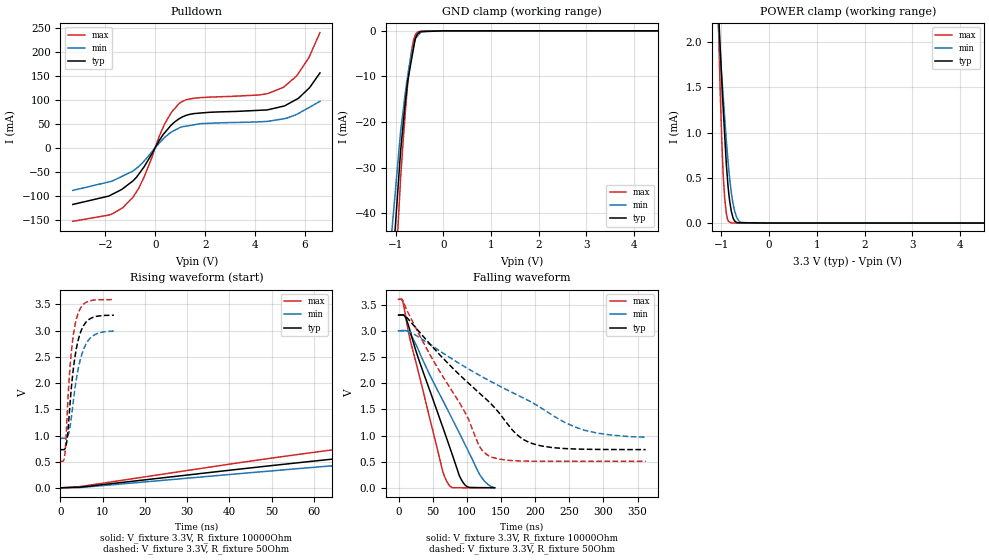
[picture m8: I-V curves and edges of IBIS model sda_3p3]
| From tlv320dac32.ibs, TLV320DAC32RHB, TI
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|   sda_3p3 Model
[Model]   sda_3p3
Model_type   I/O_open_drain
Polarity   Inverting
Vinl = 0.99
Vinh = 2.31
Vmeas = 1.65
Vref = 3.3
Cref = 10pF
Rref = 10000
|   typ   min   max
|   (nom PVT)   (fast PVT)   (slow PVT)
|C_comp from frequency sweep method (F=0.4MHz)
|C_comp   2.677e-10   2.502e-10   2.745e-10
|ON state : BUFFER OUTPUT TURNED LOW
|C_comp   5.318e-10   4.968e-10   5.453e-10
|OFF state: BUFFER IN HIGH IMPEDANCE
|C_comp   3.566e-12   3.518e-12   3.605e-12
|C_comp from LC tank measurement(L=1nH)
|Resonant Frequency(Hz)   4.560e+09   4.570e+09   4.560e+09
|C_comp   1.219e-12   1.214e-12   1.219e-12
|ON state : BUFFER OUTPUT TURNED LOW
|Resonant Frequency(Hz)   4.560e+09   4.570e+09   4.560e+09
|C_comp   1.219e-12   1.214e-12   1.219e-12
|OFF state: BUFFER IN HIGH IMPEDANCE
|Resonant Frequency(Hz)   4.780e+09   4.800e+09   4.770e+09
C_comp   1.110e-12   1.100e-12   1.114e-12
[model spec]
|subparameter   typ   min   max
Vinl   0.99   0.90   1.08
Vinh   2.31   2.10   2.52
| Where nom  PVT is Nominal Process, 3.3V, 45C
|   Fast PVT is Strong Process,  3.6V, -40C
|   Slow PVT is Weak Process,   3V, 105C
[Voltage Range]   3.3   3   3.6
|Ambient Temperature   25   85   -40
|Junction Temperature
[Temperature Range]   45   105   -40
[Pullup Reference]   3.3   3   3.6
[Pulldown Reference]   0   0   0
[Power Clamp Reference]   3.3   3   3.6
[GND Clamp Reference]   0   0   0
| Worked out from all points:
|   slope of the pulldown table from 0 to 0.495 V, typ, clamps not added: 13 ohm
|   GND clamp passes 1 mA (typ) near -0.56 V on its own axis
|   POWER clamp passes 1 mA (typ) near -0.93 V on its own axis
|   falling waveform, V_fixture 3.3V, R_fixture 10000Ohm: 20-80 % time 53.1ns typ, 68.9ns min, 41.1ns max; typ from 3.3 V to 0.004 V
|   rising waveform, V_fixture 3.3V, R_fixture 10000Ohm: 20-80 % time 454ns typ, 534ns min, 373ns max; typ from 0.003 V to 3.3 V
|   falling waveform, V_fixture 3.3V, R_fixture 50Ohm: 20-80 % time 115ns typ, 164ns min, 79.8ns max; typ from 3.3 V to 0.731 V
|   rising waveform, V_fixture 3.3V, R_fixture 50Ohm: 20-80 % time 2.17ns typ, 2.62ns min, 1.74ns max; typ from 0.731 V to 3.29 V
[Pulldown]
|   Voltage   I(typ)   I(min)   I(max)
-3.3V     -118.5mA   -89.27mA   -153.7mA
-1.696V   -96.69mA   -69.08mA   -137.7mA
-896.4mV  -69.64mA   -49.05mA   -103.7mA
-439.2mV  -39.66mA   -27.69mA   -60.66mA
381.6mV   31.19mA    21.56mA    49.68mA
1.001V    61.54mA    42.22mA    93.59mA
1.591V    71.25mA    47.97mA    103.4mA
4.162V    77.88mA    53.87mA    109.8mA
5.137V    86.55mA    60.08mA    125.8mA
5.674V    101.1mA    69.49mA    150.1mA
6.152V    123.6mA    83.47mA    187.5mA
6.6V      156mA      96.54mA    240.1mA
[GND Clamp]
|   Voltage   I(typ)   I(min)   I(max)
-3.3V     -1.343A    -1.199A    -1.533A
-1.487V   -114.4mA   -92.2mA    -146.8mA
-897.6mV  -26.39mA   -22.11mA   -32.41mA
-792mV    -15.05mA   -13.04mA   -16.99mA
-745.8mV  -10.84mA   -9.703mA   -11.43mA
-702mV    -8.268mA   -6.817mA   -7.045mA
-622.8mV  -3.616mA   -3.166mA   -1.957mA
-590.7mV  -1.731mA   -1.919mA   -1.015mA
-532.8mV  -615uA     -1.015mA   -208.3uA
-465mV    -195.4uA   -194.6uA   -64.22uA
-285mV    -119.2uA   -2.502uA   -4.665uA
6.6V      0A         0A         0A
[POWER Clamp]
|   Voltage   I(typ)   I(min)   I(max)
-3.3V     32.08mA    22.4mA     56.05mA
-1.089V   2.679mA    2.39mA     2.744mA
-1.03V    1.983mA    1.906mA    1.532mA
-993.6mV  1.586mA    1.634mA    934uA
-964.8mV  1.288mA    1.419mA    561.5uA
-932.4mV  983.8uA    1.176mA    280.4uA
-896.4mV  648.9uA    907.5uA    104uA
-864.6mV  429.3uA    705.3uA    36.05uA
-792mV    130.4uA    335uA      1.308uA
-681mV    8.006uA    64.67uA    29.88nA
-585mV    3.401uA    6.441uA    18.04nA
6.6V      0A         0A         0A
[Ramp]
R_load = 10000
|   typ   min   max
dV/dt_r   1.97707/4.5319e-07   1.79454/5.33533e-07   2.15847/3.71605e-07
dV/dt_f   1.978/5.31007e-08   1.79731/6.88447e-08   2.15865/4.1098e-08
[Falling Waveform]
V_fixture = 3.3V
V_fixture_min = 3V
V_fixture_max = 3.6V
R_fixture = 10000Ohm
|   Time   V(typ)   V(min)   V(max)
0s        3.3V       3V         3.6V
5.5ns     3.306V     3.003V     3.588V
11.5ns    3.219V     3V         3.186V
20.7ns    2.823V     2.866V     2.638V
64.9ns    1.155V     1.668V     307.9mV
70.1ns    960.6mV    1.536V     138.2mV
88.9ns    238.4mV    1.051V     2.559mV
97.1ns    59.78mV    836.1mV    1.615mV
120ns     5.102mV    230.9mV    2.415mV
140.7ns   3.888mV    754.4uV    2.291mV
[Rising Waveform]
V_fixture = 3.3V
V_fixture_min = 3V
V_fixture_max = 3.6V
R_fixture = 10000Ohm
|   Time   V(typ)   V(min)   V(max)
0s        3.332mV    4.479mV    2.252mV
69.5ns    592.5mV    457mV      780.7mV
123ns     998.6mV    784.9mV    1.286V
186.7ns   1.403V     1.12V      1.772V
254.9ns   1.759V     1.423V     2.182V
412.9ns   2.35V      1.952V     2.816V
605.5ns   2.774V     2.364V     3.221V
851.1ns   3.053V     2.664V     3.45V
1.236us   3.225V     2.877V     3.565V
2.5us     3.298V     2.995V     3.6V
[Falling Waveform]
V_fixture = 3.3V
V_fixture_min = 3V
V_fixture_max = 3.6V
R_fixture = 50Ohm
|   Time   V(typ)   V(min)   V(max)
0s        3.3V       3V         3.6V
6.2ns     3.301V     3.001V     3.575V
45.25ns   2.758V     2.745V     2.562V
98.8ns    2.043V     2.298V     1.409V
119ns     1.804V     2.147V     784.3mV
131.6ns   1.653V     2.056V     616.2mV
171.5ns   1.04V      1.789V     517.8mV
197.2ns   840.9mV    1.618V     509.9mV
270.6ns   738.8mV    1.109V     507.9mV
361.8ns   731.2mV    966.1mV    507.9mV
[Rising Waveform]
V_fixture = 3.3V
V_fixture_min = 3V
V_fixture_max = 3.6V
R_fixture = 50Ohm
|   Time   V(typ)   V(min)   V(max)
0s        730.9mV    946.2mV    507.9mV
950ps     735.9mV    946.2mV    584.6mV
1.45ns    858.8mV    955mV      1.169V
2ns       1.321V     1.059V     1.998V
2.6ns     1.923V     1.358V     2.61V
3.25ns    2.396V     1.783V     3.014V
4.1ns     2.782V     2.225V     3.309V
5.4ns     3.085V     2.625V     3.497V
6.9ns     3.22V      2.843V     3.568V
12.65ns   3.293V     2.992V     3.59V
